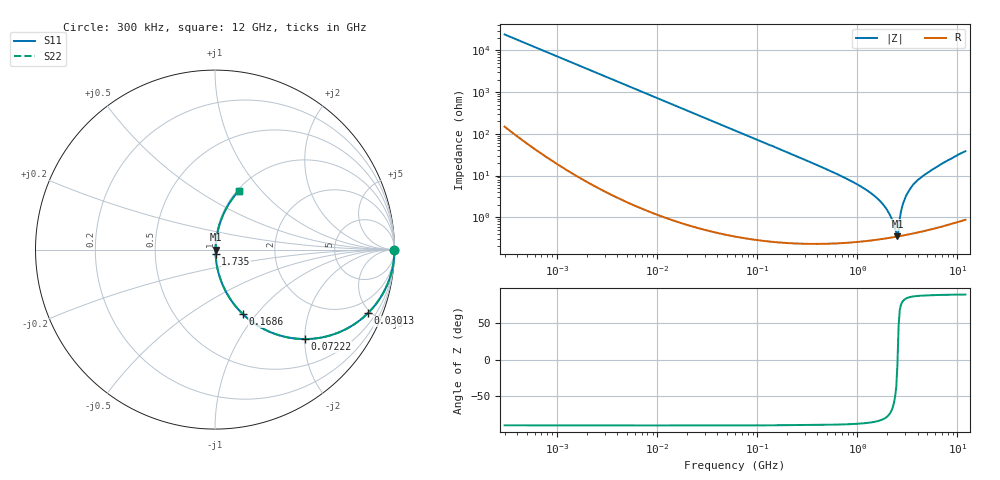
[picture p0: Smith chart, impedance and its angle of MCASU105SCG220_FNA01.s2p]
! MCASU105SCG220_FNA01  S-PARAMETER MODEL  ( General Type )
! Model Generated by TAIYO YUDEN Corporation (http://www.ty-top.com)
! Version 1.0
! TAIYO YUDEN Control No. 130207
! Copyright(c) 2013 TAIYO YUDEN CO.,LTD. All Rights Reserved.
! Product Description (link to TY-COMPAS)
! https://ds.yuden.co.jp/TYCOMPAS/or/detail?pn=MCASU105SCG220JFNA01&u=M
! Products Name : Multilayer Ceramic Capacitors
! Characteristics :
!  Capacitance : 22 pF , Rated Voltage : 50V , TCC : CG / C0G
!  Case Size : 1.0 x 0.5 / 0.039 x 0.02 [mm/inch] , Thickness : 0.5 / 0.02 [mm/inch]
!  (Conditions: Temperature = 25 degC , DC Bias Current/Voltage = 0A / 0V)
! External Node Assignments :
!  1  o---| |---o  2
! GND o---------o GND
! Frequency Range : 300000Hz  -  12GHz  [ 401 STEP ]
# MHz S RI R 50
! Freq[MHz].  S11 Real  S11 Imag  S21 Real  S21 Imag  S12 Real  S12 Imag  S22 Real  S22 Imag
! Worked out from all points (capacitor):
!   401 points, 300 kHz to 12 GHz, reference 50 ohm
!   read as one part in series: C = 22 pF near 316.3 kHz
!   lowest |Z| = 348 mohm at 2.514 GHz (marker M1)
!   series resonance near 2.521 GHz, so ESL is about 180 pH
!   S11 on the Smith chart (normalised r, x): 300 kHz: open; 30.13 MHz: 1.01, -4.80; 72.22 MHz: 1.01, -2.00; 168.6 MHz: 1.00, -0.85; 1.735 GHz: 1.01, -0.05; 12 GHz: 1.02, +0.77
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0.3  1 -0.00415  4.27e-05 0.00415  4.27e-05 0.00415  1 -0.00415
1.769972  0.9994 -0.0244  0.000647 0.0244  0.000647 0.0244  0.9994 -0.0244
10.44266  0.9794 -0.1413  0.0206 0.1413  0.0206 0.1413  0.9794 -0.1413
30.13126  0.8517 -0.3544  0.1483 0.3544  0.1483 0.3544  0.8517 -0.3544
60  0.592 -0.49  0.408 0.49  0.408 0.49  0.592 -0.49
72.22496  0.5005 -0.4984  0.4995 0.4984  0.4995 0.4984  0.5005 -0.4984
168.5979  0.1559 -0.3598  0.8441 0.3598  0.8441 0.3598  0.1559 -0.3598
353.9943  0.0407 -0.1919  0.9593 0.1919  0.9593 0.1919  0.0407 -0.1919
994.7115  0.00632 -0.0612  0.9937 0.0612  0.9937 0.0612  0.00632 -0.0612
1366.97  0.00418 -0.0376  0.9958 0.0376  0.9958 0.0376  0.00418 -0.0376
1735.023  0.00349 -0.0224  0.9965 0.0224  0.9965 0.0224  0.00349 -0.0224
2088.533  0.00332 -0.0115  0.9967 0.0115  0.9967 0.0115  0.00332 -0.0115
2384.334  0.00338 -0.00403  0.9966 0.00403  0.9966 0.00403  0.00338 -0.00403
2448.343  0.00341 -0.00259  0.9966 0.00259  0.9966 0.00259  0.00341 -0.00259
2514.07  0.00344 -0.000417  0.9966 0.000417  0.9966 0.000417  0.00344 -0.000417
2650.866  0.00359 0.00838  0.9964 -0.00838  0.9964 -0.00838  0.00359 0.00838
2795.104  0.00389 0.017  0.9961 -0.017  0.9961 -0.017  0.00389 0.017
2947.191  0.00433 0.0253  0.9957 -0.0253  0.9957 -0.0253  0.00433 0.0253
3276.641  0.00571 0.0427  0.9943 -0.0427  0.9943 -0.0427  0.00571 0.0427
3740.715  0.00845 0.0653  0.9916 -0.0653  0.9916 -0.0653  0.00845 0.0653
6354.153  0.0324 0.1611  0.9676 -0.1611  0.9676 -0.1611  0.0324 0.1611
12000  0.1334 0.3288  0.8666 -0.3288  0.8666 -0.3288  0.1334 0.3288
